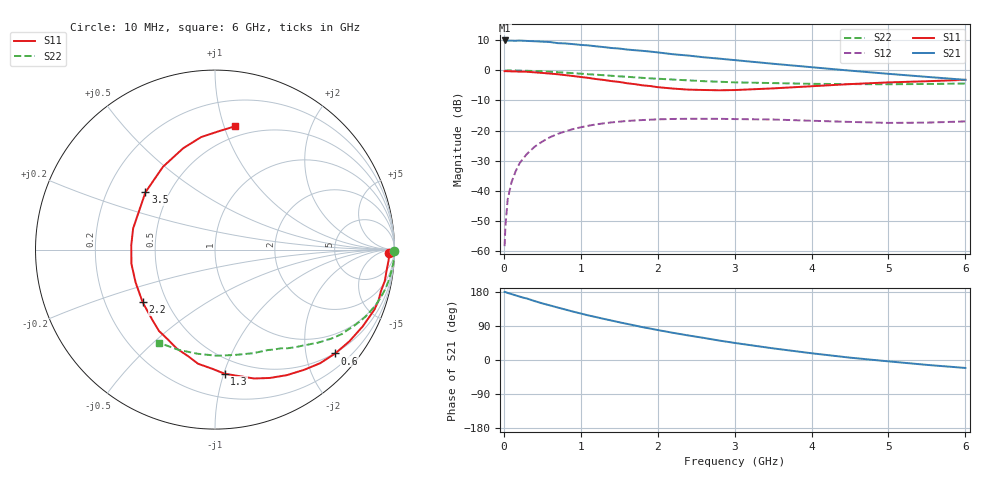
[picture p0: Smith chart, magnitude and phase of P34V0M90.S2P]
! SIEMENS Small Signal Semiconductors
! BFP181
! Si NPN RF Bipolar Junction Transistor in SOT143
! VCE = 4 V  IC = 0.9 mA
! Common Emitter S-Parameters:  March  1996
# GHz  S  MA  R  50
!  f  S11  S21  S12  S22
! GHz  MAG  ANG  MAG  ANG  MAG  ANG  MAG  ANG
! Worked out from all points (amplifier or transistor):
!   36 points, 10 MHz to 6 GHz, reference 50 ohm
!   highest |S21| = 9.9 dB at 10 MHz (marker M1)
!   |S21| within 3 dB of that: start of sweep to 1.595 GHz
!   unconditionally stable (mu >= 1): 3.276 GHz to end of sweep
!   at 250 MHz: K = 0.07, MSG = 19.6 dB, |S12| = -29.3 dB
!   at 1.4 GHz: K = 0.48, MSG = 12.4 dB, |S12| = -17.3 dB
!   at 6 GHz: K = 1.30, MAG = 3.6 dB, |S12| = -17.0 dB
!   S11 on the Smith chart (normalised r, x): 10 MHz: 49, -27; 600 MHz: 0.49, -2.61; 1.3 GHz: 0.38, -1.01; 2.2 GHz: 0.37, -0.29; 3.5 GHz: 0.37, +0.32; 6 GHz: 0.41, +1.09
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0.01  0.969 -1.0  3.143 179.5  0.0012 80.6  0.9995 -0.3
0.02  0.9722 -1.4  3.13 179.4  0.0025 91.3  0.9928 -0.6
0.05  0.9692 -3.4  3.132 177.0  0.0072 90.1  0.9965 -1.6
0.1  0.9631 -7.0  3.119 174.0  0.0139 83.9  0.998 -3.2
0.15  0.9621 -10.4  3.106 170.8  0.0205 83.1  0.9949 -4.8
0.2  0.9531 -14.1  3.133 167.7  0.028 80.9  0.9918 -6.5
0.3  0.9492 -20.6  3.085 162.3  0.0409 76.7  0.9842 -9.7
0.4  0.9278 -27.4  3.049 155.5  0.0539 71.8  0.9753 -12.7
0.6  0.8853 -40.8  2.957 144.0  0.0775 62.7  0.9488 -18.8
0.9  0.8056 -60.3  2.732 127.7  0.1059 50.8  0.8989 -26.6
1.1  0.7506 -73.1  2.6 117.6  0.1204 44.0  0.8633 -31.3
1.3  0.6936 -85.6  2.438 108.5  0.1318 37.4  0.8305 -35.7
1.5  0.6431 -98.4  2.307 99.6  0.1405 32.0  0.7964 -39.3
1.8  0.5651 -117.8  2.114 86.8  0.1496 25.0  0.7519 -44.3
2.2  0.4988 -143.9  1.854 71.7  0.1559 16.6  0.7039 -50.6
2.4  0.4788 -157.5  1.763 64.7  0.157 13.0  0.6828 -53.6
2.8  0.4672 177.1  1.568 51.3  0.1567 7.3  0.6479 -59.2
3.5  0.5022 140.5  1.289 30.7  0.1527 0.1  0.6151 -69.8
4  0.5451 122.1  1.13 17.8  0.1456 -3.0  0.5979 -78.8
4.5  0.592 107.4  0.991 6.2  0.1393 -4.7  0.5917 -88.9
5.5  0.6601 88.1  0.78 -12.9  0.1356 -1.2  0.5944 -110.0
6  0.6964 80.7  0.697 -21.0  0.142 0.3  0.6054 -120.9
